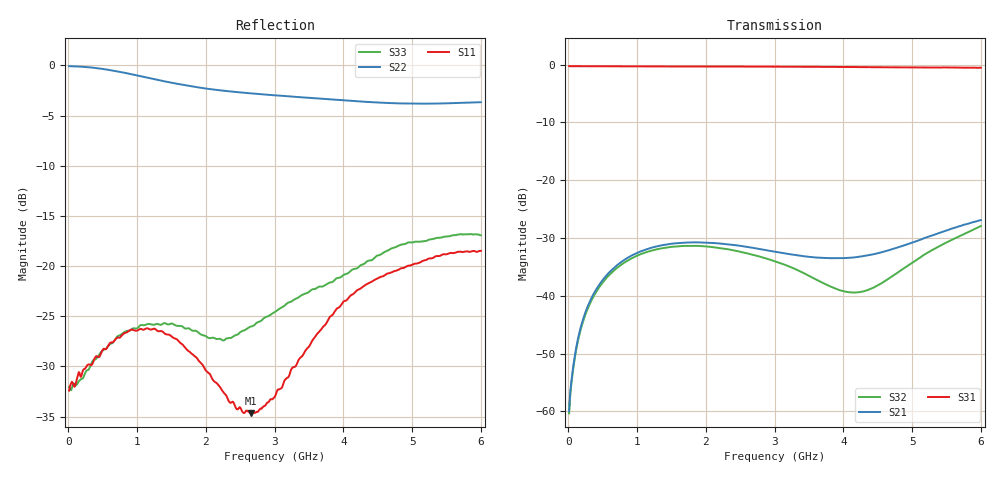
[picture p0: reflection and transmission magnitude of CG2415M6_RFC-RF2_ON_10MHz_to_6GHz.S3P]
!CEL
!CG2415M6
!Port1: RFC Port2: RF1  Port3: RF2
!Freq	S11 S12	S13 S21 S22 S23 S31 S32 S33
# Hz S dB R 50
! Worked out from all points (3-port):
!   600 points, 10 MHz to 6 GHz, reference 50 ohm
!   strongest paths, dB at 10 MHz, 1.51 GHz, 3.01 GHz, 4.51 GHz, 6 GHz:
!     S31: -0.3, -0.3, -0.4, -0.5, -0.5
!     S21: -59.9, -31.0, -32.4, -32.6, -26.9
!     S32: -60.3, -31.5, -34.0, -38.1, -27.9
!   lowest |S11| = -34.7 dB at 2.66 GHz (marker M1), VSWR 1.04, Z = 50.2 + j1.84 ohm
!   |S11| at or under -10 dB: start of sweep to end of sweep
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1e7  -32.42 1.9  -60.04 20.2  -0.29 -0.1
     -59.89 20.0  -0.08 -0.8  -60.47 19.8
     -0.28 -0.2  -60.33 20.0  -32.02 -1.3
1.1e8  -31.62 15.0  -49.17 64.7  -0.29 -1.1
       -49.18 64.9  -0.10 -7.6  -49.57 64.4
       -0.29 -1.1  -49.55 64.4  -31.89 12.5
2.4e8  -30.24 21.5  -43.08 70.5  -0.29 -2.2
       -43.08 70.4  -0.15 -16.6  -43.50 69.5
       -0.29 -2.2  -43.49 69.5  -30.74 24.9
7e8  -27.20 37.8  -34.80 60.7  -0.31 -6.2
     -34.78 60.7  -0.58 -47.5  -35.23 58.3
     -0.31 -6.2  -35.24 58.3  -27.10 40.9
1.39e9  -26.66 44.5  -31.18 42.9  -0.33 -12.0
        -31.20 42.8  -1.57 -89.4  -31.72 38.2
        -0.33 -12.0  -31.72 38.2  -25.69 42.9
1.97e9  -30.06 49.3  -30.78 33.3  -0.35 -16.8
        -30.79 33.2  -2.27 -117.9  -31.45 25.8
        -0.35 -16.9  -31.43 25.9  -26.92 27.1
2.66e9  -34.68 82.3  -31.69 29.7  -0.36 -22.7
        -31.66 29.9  -2.79 -143.7  -32.82 17.8
        -0.36 -22.8  -32.84 17.8  -26.02 -5.5
3.01e9  -32.93 98.1  -32.34 31.6  -0.37 -25.7
        -32.39 31.9  -2.98 -154.5  -34.08 17.2
        -0.37 -25.8  -34.05 17.0  -24.56 -10.2
4.25e9  -22.24 71.2  -33.18 60.6  -0.44 -36.6
        -33.21 60.7  -3.60 171.5  -39.46 65.7
        -0.44 -36.7  -39.33 65.9  -19.92 16.1
6e9  -18.48 47.4  -26.82 83.4  -0.57 -52.5
     -26.91 84.3  -3.67 128.6  -27.94 110.4
     -0.54 -52.5  -27.93 108.8  -16.93 12.2
